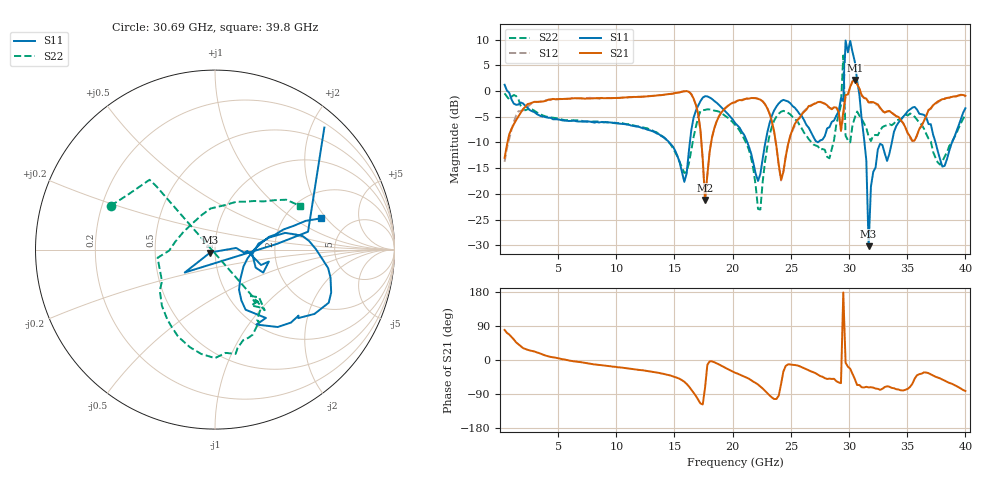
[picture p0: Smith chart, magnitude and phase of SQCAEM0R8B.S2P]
! Network Analyzer HP8722ES.07.66: Jul 25, 2000 Serial No. US39175408
! 26 Oct 2004  09:51:20
! Frequency  S11  S21  S12  S22
# HZ  S  DB R  50
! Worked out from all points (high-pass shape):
!   201 points, 400 MHz to 40 GHz, reference 50 ohm
!   highest |S21| = 2.16 dB at 30.5 GHz (marker M1); lowest = -21.2 dB at 17.63 GHz (marker M2)
!   |S21| within 3 dB of the highest: 13.58 GHz to 16.49 GHz (2.908 GHz wide, 19.3 % of centre); 29.7 GHz to 31.09 GHz (1.392 GHz wide, 4.58 % of centre)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
!   lowest |S11| = -30.1 dB at 31.68 GHz (marker M3), VSWR 1.06, Z = 47.4 - j1.54 ohm
!   |S11| at or under -10 dB: 14.55 GHz to 16.32 GHz (1.775 GHz wide, 11.5 % of centre); 21.26 GHz to 22.81 GHz (1.547 GHz wide, 7.02 % of centre); 31.32 GHz to 33.68 GHz (2.354 GHz wide, 7.24 % of centre)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
!   |S22| runs from -23.0 to 6.9 dB; largest |S21 - S12| = 0.2
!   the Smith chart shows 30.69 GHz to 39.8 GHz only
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4e8  1.21 -11.2  -12.99 79.3  -13.76 83.8  -0.46 -4.7
7.132e9  -5.95 -89.3  -1.45 -6.6  -1.48 -7.5  -5.88 -106.2
1.3666e10  -8.40 -96.4  -0.82 -34.1  -0.82 -34.5  -8.39 -151.5
1.5844e10  -17.66 -55.1  -0.06 -57.5  -0.05 -57.7  -15.92 127.5
1.6636e10  -5.22 -16.4  -1.45 -86.4  -1.44 -86.6  -9.02 17.3
1.7626e10  -1.02 -56.5  -21.16 -73.1  -21.30 -69.3  -3.67 -67.3
2.02e10  -6.19 -98.9  -2.22 -33.5  -2.10 -33.4  -6.57 -146.1
2.2378e10  -16.12 -27.9  -1.69 -70.1  -1.72 -70.4  -23.04 47.2
2.416e10  -1.97 -50.3  -17.25 -63.4  -17.39 -62.4  -4.03 -90.5
2.6932e10  -8.89 -84.5  -2.58 -32.3  -2.54 -32.8  -10.38 176.0
2.8912e10  -4.76 -23.5  -3.21 -56.0  -3.30 -56.5  -6.40 93.4
2.9308e10  -1.41 -11.3  -7.71 -61.2  -7.78 -61.5  -2.72 37.2
2.9506e10  -1.97 -12.2  -4.06 178.1  -5.12 -163.8  6.89 20.7
2.9704e10  9.82 21.8  -0.79 -7.3  -1.18 2.9  -8.70 -36.6
2.9902e10  7.51 -59.2  -0.68 -17.6  -0.78 -17.9  -9.57 25.8
3.01e10  9.73 -77.2  0.80 -23.0  0.78 -23.4  -9.99 28.7
3.0496e10  5.72 -108.7  2.16 -50.2  2.11 -50.1  -5.17 -4.2
3.0694e10  2.08 41.0  1.31 -66.0  1.34 -65.9  -4.00 157.2
3.1684e10  -30.15 -148.5  -2.23 -72.2  -2.16 -71.3  -8.82 -47.3
3.3466e10  -12.21 7.9  -3.86 -70.5  -3.98 -71.8  -6.44 -58.8
3.703e10  -6.47 -53.3  -3.35 -37.9  -3.48 -37.2  -9.81 -171.9
4e10  -3.35 13.3  -0.92 -81.8  -1.10 -82.5  -4.59 20.3
